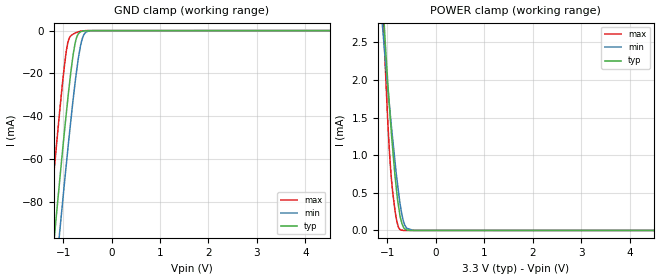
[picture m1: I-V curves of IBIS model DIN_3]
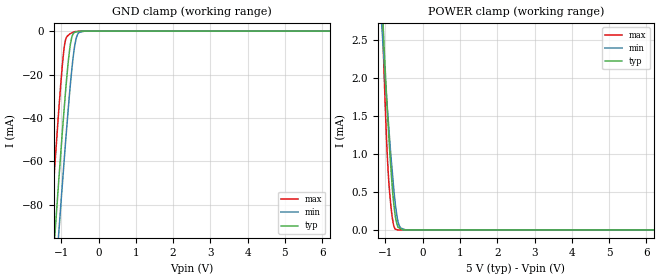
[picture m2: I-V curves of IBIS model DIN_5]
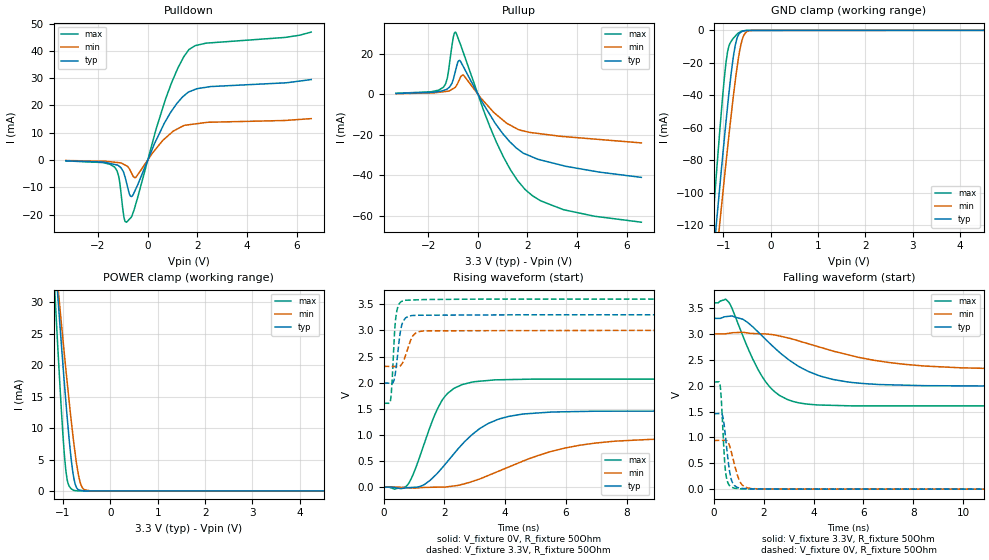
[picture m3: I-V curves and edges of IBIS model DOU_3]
|Texas Instruments Incorporated
|1- Bit, 20MHz, 2nd-Order, Isolated Delta-Sigma Modulator
| Marketing part#   Digital Voltage Range   Package-type   #pins
|AMC1204DW   3.0 to 5.5V   SOIC   16
|AMC1204DWR   3.0 to 5.5V   SOIC   16
[IBIS Ver]   4.0
[File name]   amc1204.ibs
[File Rev]   1.0
[Date]   01/25/2011
[Source]   Texas Instruments Incorporated.
   Analog-eLab, HPA
   12500 TI Blvd
   Dallas, TX -75243
   For Support e-mail: elab_ibis@list.ti.com
[Notes]   Revision History:
   1.0: 01/25/2010
   - Initial version of the model
   - Initial Model generated from simulations in TISPICED
   - Model names with a trailing _3 contains the model for
   3.3V (3.0, V and 3.6V).
   _ Model names with trailing _5 contains
   the model for 5V (4.5V and 5.5V) operation.
   - Model not matched to measurements
   - C_comp although listed in numerical order of value are
   obtained from varying PVT conditions. For PVT conditions
   for each specific value refer the buffer description under
   respective [Model]. IBIS model user is responsible for using
   appropriate C_comp to simulate for Signal Integrity.
[Disclaimer]
 This product is designed as an aid for customers of Texas Instruments.
 No warranties, either expressed or implied, with respect to this third
 party software (if any) or with respect to its fitness for any
 particular purpose is claimed by Texas Instruments or the author. The
 software (if any) is provided solely on an "as is" basis. The entire
 risk as to its quality and performance is with the customer
[Copyright] (C) Copyright 2011 Texas Instruments Incorporated.
   All rights reserved.
|   AMC1204
[Component]   amc1204dw
[Manufacturer] TI
[Package]   | 16 SOIC - DW package   9
| variable   typ   min   max
R_pkg  8.69825E-02   5.75700E-02   1.17750E-01
L_pkg  3.36294E+00nH 2.60709E+00nH 4.68074E+00nH
C_pkg  8.77755E-01pF 7.69630E-01pF 1.06049E+00pF
|-------------------------PIN------------------------------------------------
[Pin] signal_name  model_name  R_pin  L_pin C_pin
1   VDD1   POWER 0.04664  4.63776nH  1.26722pF
2   VINP   TERM  0.11775  4.68074nH  1.06049pF
3   VINM   TERM  0.09485  3.28575nH  0.76963pF
4   GND1   GND   0.00484  1.62219nH  0.70855pF
5   NC   NC   0.00484  1.62199nH  0.70856pF
6   NC   NC   0.00496  1.65136nH  0.68405pF
7   NC   NC   0.00492  1.65845nH  0.67566pF
8   GND1   GND   0.03117  4.10414nH  1.37395pF
9   GND2   GND   0.03905  4.03377nH  1.37493pF
10  NC   NC   0.10074  3.41449nH  0.78630pF
11  DATA   DOU   0.05757  2.60709nH  0.89494pF
12  NC   NC   0.00484  1.62202nH  0.70851pF
13  CLKIN   DIN   0.07776  2.87819nH  0.78596pF
14  VDD2   POWER 0.05498  3.02275nH  0.82076pF
15  NC   NC   0.00757  2.60433nH  0.94964pF
16  GND2   GND   0.01000  3.42148nH  1.17122pF
|   Model Selectors
[Model Selector]  DIN
DIN_3   3.3V digital input
DIN_5   5V digital input
|NOTES   Model DIN split into two Models DIN_3 and DIN_5
|   to accomodate voltage range of 3.0V - 5.5V
|   DIN_3 operates in voltage range of 3 - 3.3 - 3.6
|   DIN_5 operates in voltage range of 4.5 - 5 - 5.5
|   The max pin frequency for Model DIN is 24MHz.Also the
|   voltage range and frequency is referenced with datasheet.
[Model Selector]  DOU
DOU_3  3.3V digital output
DOU_5  5V digital output
|NOTES   Model DOU split into two Models DOU_3 and DOU_5
|   to accomodate voltage range of 3.0V - 5.5V
|   DOU_3 operates in voltage range of 3 - 3.3 - 3.6
|   DOU_5 operates in voltage range of 4.5 - 5 - 5.5
|   The max pin frequency for Model DOU is 12MHz.Also the
|   voltage range and frequency is referenced with datasheet.
[Model Selector]  TERM
TERM_3  3.3V digital output
TERM_5  5V digital output
|   TERM Model
[Model] TERM_3
Model_type Terminator
C_comp   1E-20   1E-20   1E-20
| variable   typ   min   max
[Voltage Range]   3.3V   3.0V   3.6V
[POWER Clamp Reference]  3.3V   2.0V   5.5V
[GND Clamp Reference]   0.0V   0.0V   0.0V
|Operating Temperature
[Temperature Range]   72   150   -40
|   TERM Model
[Model] TERM_5
Model_type Terminator
C_comp   1E-20   1E-20   1E-20
| variable   typ   min   max
[Voltage Range]   5V   4.5V   5.5V
[POWER Clamp Reference]  3.3V   2.0V   5.5V
[GND Clamp Reference]   0.0V   0.0V   0.0V
|Operating Temperature
[Temperature Range]   72   150   -40
| Models and submodels in the file (6): DIN_3 (Input), DIN_5 (Input), DOU_3 (Output), DOU_5 (Output), TERM_3 (Terminator), TERM_5 (Terminator)
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|NOTES   Model DOU split into two Models TERM_3 and TERM_5
|   to accomodate voltage range of 3.0V - 5.5V
|   TERM_3 operates in voltage range of 3 - 3.3 - 3.6
|   TERM_5 operates in voltage range of 4.5 - 5 - 5.5
|   The max pin frequency for Model DOU is 12MHz.Also the
|   voltage range and frequency is referenced with datasheet.
|   3.3 V DIN Model
[Model] DIN_3
Model_type Input
Vinl = 0.99
Vinh = 2.31
|   typ   min   max
|   (nom PVT)   (Fast PVT)   (slow PVT)
C_comp   5.83507E-13   5.37082E-13   6.3002E-13
| Where   nom PVT is  Nominal Process, 3.3V, 72C
|   Fast PVT is Strong Process, 3.6V, -40C
|   Slow PVT is Weak Process, 3.0V, 150C
|C_comp - from L-C Tank method, L = 1nH, peak frequency
| variable   typ   min   max
[Voltage Range]   3.3   3   3.6
[Temperature Range]   72   150   -40
|Operating Temperature   27   105   -40
[Power Clamp Reference]   3.3   3   3.6
[GND Clamp Reference]   0   0   0
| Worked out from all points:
|   GND clamp passes 1 mA (typ) near -0.67 V on its own axis
|   POWER clamp passes 1 mA (typ) near -0.88 V on its own axis
[GND Clamp]
|   Voltage   I(typ)   I(min)   I(max)
-3.3V     -644.6mA   -659.4mA   -624.1mA
-1.311V   -128.4mA   -151.9mA   -96.76mA
-1.199V   -100.6mA   -124.5mA   -68.47mA
-1.145V   -87.34mA   -111.5mA   -55.01mA
-1.076V   -70.72mA   -94.84mA   -38.34mA
-933.9mV  -38.22mA   -62.05mA   -9.279mA
-881.7mV  -27.13mA   -50.4mA    -3.843mA
-800mV    -12.06mA   -33.13mA   -1.73mA
-726.1mV  -3.492mA   -19.34mA   -865.1uA
-602.3mV  -290uA     -3.523mA   -172.3uA
-470.2mV  -16.89uA   -168.6uA   -17.53uA
6.59V     0A         0A         0A
[POWER Clamp]
|   Voltage   I(typ)   I(min)   I(max)
-3.3V     32.89mA    26.87mA    43.23mA
-1.101V   3.122mA    2.706mA    3.06mA
-1.047V   2.53mA     2.301mA    2.227mA
-989.1mV  1.933mA    1.876mA    1.411mA
-953.6mV  1.606mA    1.632mA    1.003mA
-916.3mV  1.281mA    1.374mA    677.7uA
-890.2mV  1.078mA    1.21mA     506.1uA
-817.7mV  572.8uA    757.7uA    163.8uA
-735.3mV  180.8uA    342.1uA    10.06uA
-640.8mV  21.85uA    70.81uA    731.5nA
-462.5mV  914.4nA    774.5nA    713.5nA
6.59V     0A         0A         0A
|   5 V DIN Model
[Model] DIN_5
Model_type Input
Vinl = 1.5
Vinh = 3.5
|   typ   min   max
|   (nom PVT)   (Fast PVT)   (slow PVT)
C_comp   5.54701E-13   5.20141E-13   5.99957E-13
| Where   nom PVT is  Nominal Process, 3.3V, 72C
|   Fast PVT is Strong Process, 3.6V, -40C
|   Slow PVT is Weak Process, 3.0V, 150C
|C_comp - from L-C Tank method, L = 1nH, peak frequency
| variable   typ   min   max
[Voltage Range]   5   4.5   5.5
[Temperature Range]   72   150   -40
|Operating Temperature   27   105   -40
[Power Clamp Reference]   5   4.5   5.5
[GND Clamp Reference]   0   0   0
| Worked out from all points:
|   GND clamp passes 1 mA (typ) near -0.67 V on its own axis
|   POWER clamp passes 1 mA (typ) near -0.88 V on its own axis
[GND Clamp]
|   Voltage   I(typ)   I(min)   I(max)
-5V       -1.093A    -1.102A    -1.081A
-1.31V    -127.9mA   -151.3mA   -96.34mA
-1.275V   -119.3mA   -142.9mA   -87.46mA
-1.164V   -92.1mA    -116.1mA   -59.76mA
-1.06V    -66.89mA   -91.15mA   -34.61mA
-970.5mV  -46.22mA   -70.42mA   -15.53mA
-911.9mV  -33.53mA   -57.18mA   -6.403mA
-773.1mV  -8.205mA   -27.86mA   -1.391mA
-651.4mV  -726.5uA   -8.112mA   -308.4uA
-555.8mV  -269uA     -1.317mA   -93uA
-370.6mV  -11.11uA   -13.06uA   -13.61uA
9.985V    0A         0A         0A
[POWER Clamp]
|   Voltage   I(typ)   I(min)   I(max)
-5V       56.62mA    46.48mA    74.97mA
-1.094V   3.055mA    2.653mA    2.965mA
-1.06V    2.667mA    2.395mA    2.412mA
-1.049V   2.545mA    2.314mA    2.246mA
-960.2mV  1.663mA    1.681mA    1.072mA
-892.9mV  1.097mA    1.229mA    522uA
-838.9mV  707.4uA    892.3uA    247.5uA
-783.8mV  375.8uA    576.8uA    67.15uA
-680.8mV  61.87uA    153uA      910.6nA
-599.4mV  18.79uA    27.57uA    903.7nA
-459.6mV  636nA      711.4nA    891.8nA
9.985V    0A         0A         0A
|   3.3 V DOU Model
[Model] DOU_3
Model_type Output
Polarity   Non-Inverting
Enable   Active-Low
Vmeas = 1.65
Vref = 1.65
Cref = 15pF
Rref = 50
|   typ   min   max
|   (nom PVT)   (Fast PVT)   (slow PVT)
|   Output high
C_comp   1.33446E-12   1.08644E-12   1.65973E-12
|   Output low
|C_comp   1.45887E-12   1.13766E-12   1.79734E-12
|   High Impedance
|C_comp   1.3308E-12   1.04622E-12   1.63671E-12
| Where   nom PVT is  Nominal Process, 3.3V, 72C
|   Fast PVT is Strong Process, 3.6V, -40C
|   Slow PVT is Weak Process, 3.0V, 150C
|C_comp - from L-C Tank method, L = 1nH, peak frequency
| variable   typ   min   max
[Voltage Range]   3.3   3   3.6
[Temperature Range]   72   150   -40
|Operating Temperature   27   105   -40
[Pullup Reference]   3.3   3   3.6
[Pulldown Reference]   0   0   0
[Power Clamp Reference]   3.3   3   3.6
[GND Clamp Reference]   0   0   0
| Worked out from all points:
|   slope of the pulldown table from 0 to 0.495 V, typ, clamps not added: 48.2 ohm
|   slope of the pullup table from 0 to 0.495 V, typ, clamps not added: 47.7 ohm
|   GND clamp passes 1 mA (typ) near -0.62 V on its own axis
|   POWER clamp passes 1 mA (typ) near -0.74 V on its own axis
|   falling waveform, V_fixture 3.3V, R_fixture 50Ohm: 20-80 % time 2.13ns typ, 3.57ns min, 1.22ns max; typ from 3.3 V to 1.99 V
|   rising waveform, V_fixture 0V, R_fixture 50Ohm: 20-80 % time 1.48ns typ, 2.71ns min, 832ps max; typ from 0 V to 1.46 V
|   rising waveform, V_fixture 3.3V, R_fixture 50Ohm: 20-80 % time 167ps typ, 252ps min, 116ps max; typ from 1.99 V to 3.3 V
|   falling waveform, V_fixture 0V, R_fixture 50Ohm: 20-80 % time 220ps typ, 324ps min, 145ps max; typ from 1.46 V to 0 V
[Pulldown]
|   Voltage   I(typ)   I(min)   I(max)
-3.3V     -276uA     -174.7uA   -310.5uA
-1.335V   -1.618mA   -793.7uA   -2.569mA
-1.164V   -2.159mA   -955.7uA   -6.139mA
-962.4mV  -4.743mA   -1.581mA   -20.66mA
-854.2mV  -8.244mA   -2.111mA   -22.76mA
-700.6mV  -13.14mA   -3.853mA   -21.32mA
-597.7mV  -12.87mA   -5.733mA   -19.51mA
-468.7mV  -10.38mA   -6.272mA   -15.75mA
714.2mV   14.2mA     8.048mA    22.19mA
1.212V    21.1mA     11.47mA    33.6mA
1.655V    24.95mA    12.93mA    40.37mA
6.59V     29.48mA    15.17mA    46.86mA
[GND Clamp]
|   Voltage   I(typ)   I(min)   I(max)
-3.3V     -854.8mA   -807.5mA   -982.9mA
-1.228V   -146.1mA   -164.3mA   -121mA
-1.147V   -119.9mA   -140.5mA   -89.51mA
-1.075V   -97.21mA   -119.6mA   -62.65mA
-978.3mV  -67.18mA   -91.81mA   -29.76mA
-913mV    -48.1mA    -73.76mA   -14.01mA
-835.9mV  -27.27mA   -53.18mA   -6.994mA
-747.4mV  -9.298mA   -31.42mA   -3.602mA
-622.1mV  -955uA     -8.256mA   -589.6uA
-537.2mV  -229.6uA   -1.766mA   -127.5uA
-367.5mV  -28.6uA    -26.1uA    -47.17uA
6.59V     0A         0A         0A
[Pullup]
|   Voltage   I(typ)   I(min)   I(max)
-3.3V     351uA      257.1uA    421.6uA
-1.39V    1.827mA    1.197mA    3.39mA
-1.232V   2.604mA    1.424mA    7.838mA
-996.1mV  7.089mA    2.727mA    27.56mA
-904.4mV  11.28mA    3.437mA    30.63mA
-738.6mV  16.7mA     7.302mA    25.8mA
-579.6mV  13.51mA    9.355mA    20.38mA
726.6mV   -14.81mA   -9.85mA    -23.05mA
1.317V    -23.79mA   -15.34mA   -37.31mA
1.893V    -29.4mA    -18.28mA   -46.83mA
3.427V    -35.19mA   -20.86mA   -56.86mA
6.59V     -41.03mA   -24.03mA   -63.13mA
[POWER Clamp]
|   Voltage   I(typ)   I(min)   I(max)
-3.3V     278.5mA    226.3mA    361.9mA
-1.174V   37.71mA    37.94mA    31.86mA
-1.164V   36.7mA     37.16mA    30.51mA
-1.107V   30.78mA    32.52mA    22.51mA
-1.074V   27.28mA    29.84mA    18.02mA
-1.006V   20.5mA     24.46mA    9.447mA
-938.7mV  14.13mA    19.29mA    3.166mA
-888.7mV  9.781mA    15.62mA    1.1mA
-772.6mV  2.102mA    7.674mA    86.09uA
-624.6mV  108.5uA    1.065mA    6.534uA
-422.2mV  5.179uA    6.189uA    6.351uA
6.59V     0A         0A         0A
[Ramp]
R_load = 50
|   typ   min   max
dV/dt_r   0.874562/1.47446e-009  0.563757/2.69542e-009   1.24145/8.32032e-010
dV/dt_f   0.784539/2.11034e-009  0.412963/3.55876e-009   1.19615/1.22231e-009
[Falling Waveform]
V_fixture = 3.3V
V_fixture_min = 3V
V_fixture_max = 3.6V
R_fixture = 50Ohm
C_fixture = 0F
|   Time   V(typ)   V(min)   V(max)
0s        3.3V       3V         3.6V
471.5ps   3.332V     3.002V     3.672V
591.2ps   3.339V     3.01V      3.617V
1.177ns   3.279V     3.03V      2.948V
2.03ns    2.917V     2.999V     2.109V
2.616ns   2.652V     2.961V     1.818V
3.357ns   2.386V     2.871V     1.673V
5.32ns    2.074V     2.604V     1.612V
8.422ns   2V         2.38V      1.609V
19.63ns   1.992V     2.312V     1.606V
[Rising Waveform]
V_fixture = 0V
V_fixture_min = 0V
V_fixture_max = 0V
R_fixture = 50Ohm
C_fixture = 0F
|   Time   V(typ)   V(min)   V(max)
0s        2.038nV    5.064nV    1.683nV
780.9ps   -11.01mV   -11.86mV   38.03mV
1.331ns   47.06mV    -6.028mV   823.4mV
1.909ns   357.9mV    620.9uV    1.647V
2.311ns   636.3mV    22.13mV    1.889V
2.917ns   1.008V     108.3mV    2.011V
3.761ns   1.297V     299.1mV    2.054V
4.528ns   1.394V     483.8mV    2.063V
7.512ns   1.454V     874.1mV    2.067V
19.63ns   1.458V     939.6mV    2.069V
[Rising Waveform]
V_fixture = 3.3V
V_fixture_min = 3V
V_fixture_max = 3.6V
R_fixture = 50Ohm
C_fixture = 0F
|   Time   V(typ)   V(min)   V(max)
0s        1.992V     2.312V     1.606V
220.5ps   1.99V      2.31V      1.645V
262ps     1.989V     2.309V     1.879V
328.1ps   2.023V     2.309V     2.608V
410ps     2.284V     2.308V     3.289V
558.9ps   3.008V     2.326V     3.541V
692ps     3.217V     2.473V     3.576V
965.3ps   3.286V     2.899V     3.583V
1.361ns   3.291V     2.992V     3.591V
19.63ns   3.3V       3V         3.6V
[Falling Waveform]
|Gnd
V_fixture = 0V
V_fixture_min = 0V
V_fixture_max = 0V
R_fixture = 50Ohm
C_fixture = 0F
|   Time   V(typ)   V(min)   V(max)
0s        1.458V     939.6mV    2.069V
258.4ps   1.462V     942.9mV    1.991V
367.7ps   1.391V     944.3mV    1.127V
437.7ps   1.152V     945.1mV    520.5mV
506.8ps   846.8mV    941mV      227.4mV
642.3ps   320mV      822.9mV    64.26mV
823.7ps   73.61mV    489mV      18.46mV
1.133ns   14.02mV    83.55mV    4.887mV
1.55ns    5.282mV    10.17mV    3.588mV
19.63ns   22.61nV    1.296uV    4.588nV
